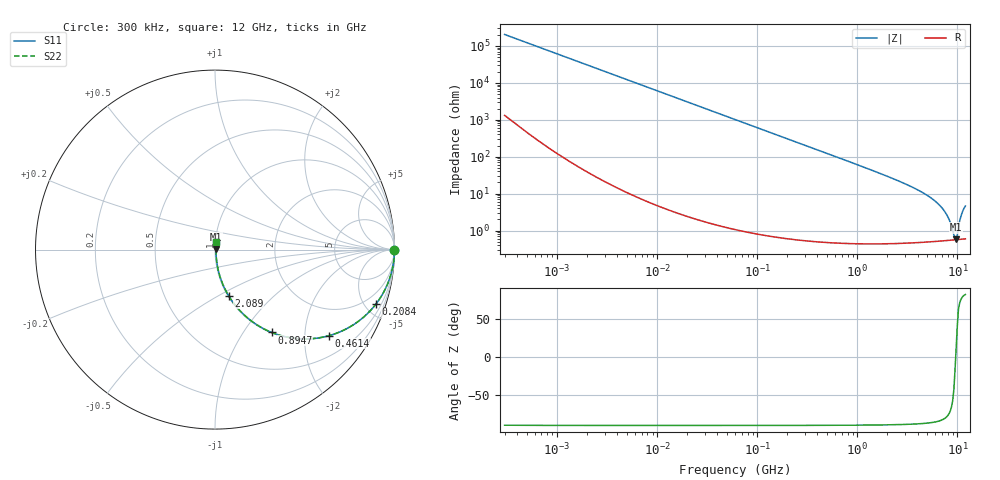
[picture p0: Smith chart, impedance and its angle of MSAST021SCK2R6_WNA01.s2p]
! MSAST021SCK2R6_WNA01  S-PARAMETER MODEL  ( General Type )
! Model Generated by TAIYO YUDEN Corporation (http://www.ty-top.com)
! Version 2.0
! TAIYO YUDEN Control No. 181101
! Copyright(c) 2015 TAIYO YUDEN CO.,LTD. All Rights Reserved.
! Product Description (link to TY-COMPAS)
! https://ds.yuden.co.jp/TYCOMPAS/or/detail?pn=MSAST021SCK2R6BWNA01&u=M
! Products Name : Multilayer Ceramic Capacitors
! Characteristics :
!  Capacitance : 2.6 pF , Rated Voltage : 25V , TCC : CK / C0K
!  Case Size : 0.25 x 0.125 / 0.0098 x 0.0049 [mm/inch] , Thickness : 0.125 / 0.0049 [mm/inch]
!  (Conditions: Temperature = 25 degC , DC Bias Current/Voltage = 0A / 0V)
! External Node Assignments :
!  1  o---| |---o  2
! GND o---------o GND
! Frequency Range : 0.3MHz  -  12000MHz  [ 401 STEP ]
# MHz S RI R 50
! Freq[MHz].  S11 Real  S11 Imag  S21 Real  S21 Imag  S12 Real  S12 Imag  S22 Real  S22 Imag
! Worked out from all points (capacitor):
!   401 points, 300 kHz to 12 GHz, reference 50 ohm
!   read as one part in series: C = 2.6 pF near 316.3 kHz
!   lowest |Z| = 580 mohm at 9.708 GHz (marker M1)
!   series resonance near 9.593 GHz, so ESL is about 110 pH
!   S11 on the Smith chart (normalised r, x): 300 kHz: open; 208.4 MHz: 1.01, -5.87; 461.4 MHz: 1.01, -2.65; 894.7 MHz: 1.01, -1.36; 2.089 GHz: 1.01, -0.56; 12 GHz: 1.01, +0.09
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0.3  1 -0.00049  3.4e-06 0.00049  3.4e-06 0.00049  1 -0.00049
1.769972  1 -0.00289  1.23e-05 0.00289  1.23e-05 0.00289  1 -0.00289
10.44266  0.9997 -0.0171  0.000304 0.0171  0.000304 0.0171  0.9997 -0.0171
60  0.9904 -0.0971  0.00962 0.0971  0.00962 0.0971  0.9904 -0.0971
208.3979  0.8956 -0.3048  0.1044 0.3048  0.1044 0.3048  0.8956 -0.3048
353.9943  0.7482 -0.4326  0.2518 0.4326  0.2518 0.4326  0.7482 -0.4326
461.3684  0.6362 -0.4793  0.3638 0.4793  0.3638 0.4793  0.6362 -0.4793
634.0297  0.4803 -0.4973  0.5197 0.4973  0.5197 0.4973  0.4803 -0.4973
894.6982  0.3162 -0.4618  0.6838 0.4618  0.6838 0.4618  0.3162 -0.4618
1366.97  0.1638 -0.3652  0.8362 0.3652  0.8362 0.3652  0.1638 -0.3652
2088.533  0.0758 -0.2569  0.9242 0.2569  0.9242 0.2569  0.0758 -0.2569
3944.255  0.0208 -0.1256  0.9792 0.1256  0.9792 0.1256  0.0208 -0.1256
6026.253  0.00872 -0.0605  0.9913 0.0605  0.9913 0.0605  0.00872 -0.0605
6879.757  0.00699 -0.0426  0.993 0.0426  0.993 0.0426  0.00699 -0.0426
7648.807  0.00611 -0.0287  0.9939 0.0287  0.9939 0.0287  0.00611 -0.0287
8281.503  0.00572 -0.0185  0.9943 0.0185  0.9943 0.0185  0.00572 -0.0185
9207.246  0.00555 -0.00501  0.9945 0.00501  0.9945 0.00501  0.00555 -0.00501
9454.42  0.00556 -0.00166  0.9944 0.00166  0.9944 0.00166  0.00556 -0.00166
9708.23  0.0056 0.00138  0.9944 -0.00138  0.9944 -0.00138  0.0056 0.00138
9968.853  0.00566 0.00501  0.9943 -0.00501  0.9943 -0.00501  0.00566 0.00501
11083.22  0.0066 0.0284  0.9934 -0.0284  0.9934 -0.0284  0.0066 0.0284
12000  0.00796 0.0451  0.992 -0.0451  0.992 -0.0451  0.00796 0.0451
